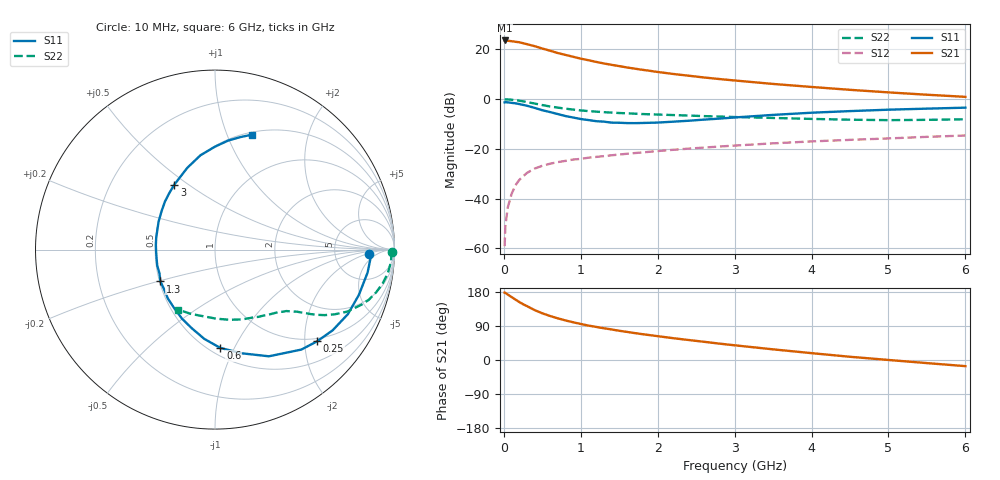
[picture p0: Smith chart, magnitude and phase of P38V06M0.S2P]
! SIEMENS Small Signal Semiconductors
! BFP181
! Si NPN RF Bipolar Junction Transistor in SOT143
! VCE = 8 V  IC = 6 mA
! Common Emitter S-Parameters:  March  1996
# GHz  S  MA  R  50
!  f  S11  S21  S12  S22
! GHz  MAG  ANG  MAG  ANG  MAG  ANG  MAG  ANG
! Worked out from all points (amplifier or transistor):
!   36 points, 10 MHz to 6 GHz, reference 50 ohm
!   highest |S21| = 23.6 dB at 10 MHz (marker M1)
!   |S21| within 3 dB of that: start of sweep to 473.2 MHz
!   unconditionally stable (mu >= 1): 1.697 GHz to end of sweep
!   at 250 MHz: K = 0.23, MSG = 26.8 dB, |S12| = -31.1 dB
!   at 1.4 GHz: K = 0.92, MSG = 18.2 dB, |S12| = -22.6 dB
!   at 6 GHz: K = 1.05, MAG = 6.4 dB, |S12| = -14.6 dB
!   S11 on the Smith chart (normalised r, x): 10 MHz: 13, -3; 250 MHz: 0.93, -2.29; 600 MHz: 0.56, -0.88; 1.3 GHz: 0.51, -0.21; 3 GHz: 0.50, +0.44; 6 GHz: 0.53, +1.23
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0.01  0.8609 -1.7  15.12 177.8  0.0011 85.9  0.988 -0.7
0.02  0.8673 -3.5  14.97 177.1  0.0028 85.2  0.9831 -1.5
0.05  0.8596 -8.6  14.91 172.8  0.0065 85.4  0.9832 -4.0
0.1  0.8404 -17.5  14.61 166.2  0.0123 78.1  0.9713 -7.9
0.2  0.7951 -34.4  13.93 153.1  0.0236 72.5  0.9285 -14.9
0.25  0.7649 -41.9  13.31 147.2  0.0279 68.0  0.9012 -18.1
0.3  0.7359 -49.2  12.73 142.3  0.0327 64.6  0.872 -20.6
0.4  0.666 -63.2  11.6 131.7  0.04 59.4  0.8143 -25.1
0.5  0.5968 -75.5  10.39 123.2  0.0456 54.0  0.7581 -28.4
0.6  0.5487 -86.9  9.416 116.2  0.0501 51.1  0.711 -30.9
0.7  0.5007 -96.9  8.447 110.0  0.054 48.7  0.6741 -32.6
0.8  0.4563 -106.6  7.755 104.5  0.0571 47.3  0.6427 -34.0
0.9  0.4262 -115.6  7.105 99.6  0.0608 45.8  0.6148 -35.1
1.1  0.3788 -133.8  6.055 90.8  0.0663 43.9  0.5735 -37.1
1.3  0.352 -149.7  5.207 83.8  0.0712 42.5  0.5457 -39.0
1.7  0.3283 -178.7  4.097 71.1  0.0821 41.1  0.5091 -42.9
2.2  0.3512 153.4  3.205 57.6  0.0954 39.0  0.4774 -48.6
3  0.427 122.1  2.368 38.8  0.1161 34.7  0.4356 -60.0
3.5  0.4811 108.7  2.019 28.1  0.1288 31.7  0.4174 -68.7
4.5  0.5735 90.0  1.536 8.5  0.1513 24.6  0.385 -88.9
5.5  0.6425 77.3  1.224 -8.2  0.1739 18.4  0.3825 -110.5
6  0.6724 72.2  1.11 -16.2  0.1853 14.8  0.3926 -121.7
